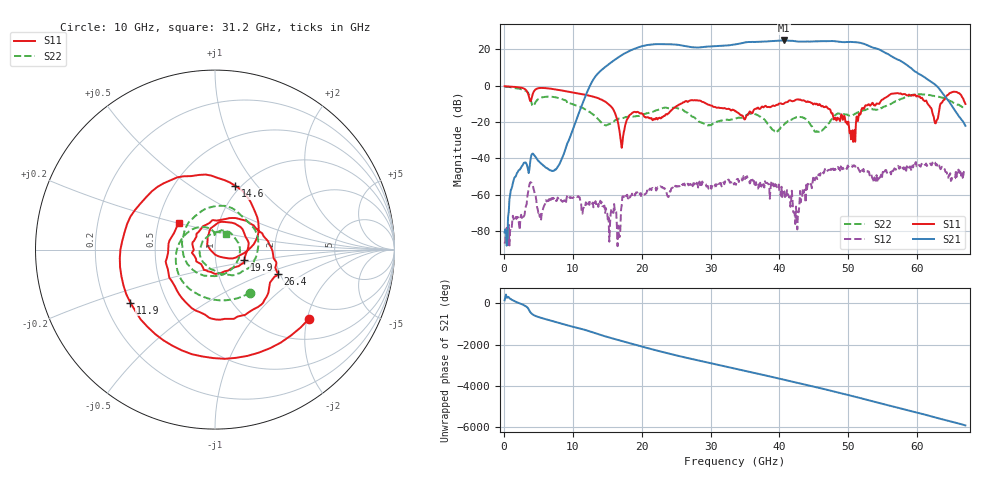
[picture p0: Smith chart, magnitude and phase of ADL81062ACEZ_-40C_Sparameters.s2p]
! Analog Devices Inc.
! Device:  ADL8106ACEZ
! Description: GaAs pHEMT Low Noise Amplifier.
! Frequency:  18.00 -  54.00 GHz
! Package:
! Conditions:	Vdd = 3.0 V
!		Idd = 120 mA
!		Temp = -40 C
! Calibration: Board loss de-embedded from S21 magnitude. All other RF measurements reference to RF coaxial connector
! Misc:DB
! Freq(GHz)	S11a(dB)	S11p(deg)	S21a(dB)	S21p(deg)	S12a(dB)	S12p(deg)	S22a(dB)	S22p(deg)
# GHz S  dB  R 50
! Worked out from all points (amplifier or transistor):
!   670 points, 100 MHz to 67 GHz, reference 50 ohm
!   highest |S21| = 24.9 dB at 40.6 GHz (marker M1)
!   |S21| within 3 dB of that: 31.22 GHz to 53.03 GHz (21.81 GHz wide, 51.8 % of centre)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
!   unconditionally stable (mu >= 1): start of sweep to end of sweep
!   at 11.2 GHz: K = 1986.18, MAG = -9.7 dB, |S12| = -64.4 dB
!   at 33.6 GHz: K = 17.39, MAG = 23.0 dB, |S12| = -54.0 dB
!   at 67 GHz: K = 1041.88, MAG = -21.3 dB, |S12| = -45.8 dB
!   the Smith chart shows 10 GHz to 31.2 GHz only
!   S11 on the Smith chart (normalised r, x): 10 GHz: 1.53, -2.05; 11.9 GHz: 0.31, -0.26; 14.6 GHz: 0.95, +0.78; 19.9 GHz: 1.38, -0.17; 26.4 GHz: 1.95, -0.63; 31.2 GHz: 0.64, +0.21
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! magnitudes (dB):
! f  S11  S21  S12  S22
! 100 MHz  -0.3  -80.8  -86.9  -0.6
! 2.2 GHz  -0.9  -46.4  -76.7  -1.7
! 3.9 GHz  -8.5  -39.7  -53.1  -8.0
! 5.3 GHz  -1.2  -42.5  -70.8  -6.7
! 7.5 GHz  -2.1  -46.3  -62.2  -6.4
! 10 GHz  -3.7  -24.2  -61.9  -10.2
! 11.3 GHz  -4.6  -10.9  -69.7  -11.9
! 11.9 GHz  -5.1  -5.1  -64.2  -13.2
! 14.6 GHz  -8.6  10.0  -66.0  -21.6
! 17.1 GHz  -34.2  16.8  -65.9  -17.9
! 19.9 GHz  -15.2  21.6  -60.8  -16.3
! 22.4 GHz  -18.0  22.9  -56.1  -13.3
! 26.4 GHz  -8.5  21.7  -54.6  -14.4
! 31.2 GHz  -12.0  21.9  -54.1  -19.5
! 33.6 GHz  -14.1  22.8  -54.0  -18.2
! 40.6 GHz  -10.0  24.9  -57.4  -21.7
! 42.5 GHz  -7.6  24.4  -73.3  -17.3
! 44.7 GHz  -9.4  24.3  -56.4  -22.2
! 50.7 GHz  -30.9  24.0  -44.2  -16.0
! 55.9 GHz  -5.3  17.2  -47.0  -10.6
! 62.7 GHz  -20.7  0.3  -43.8  -5.8
! 67 GHz  -10.1  -22.1  -45.8  -11.8
